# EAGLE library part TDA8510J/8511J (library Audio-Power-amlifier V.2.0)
The TDA8510J is an integrated class-B output amplifier in a 17-lead single-in-line (SIL) power package. It contains a 26 W Bridge-Tied Load (BTL) amplifier and 2 ´ 13 W Single-Ended (SE) amplifiers. The TDA8511J is an integrated class-B output amplifier in a 17-lead DIL-bent-SIL power package. It contains 4 ´ 13 W single-ended amplifiers.
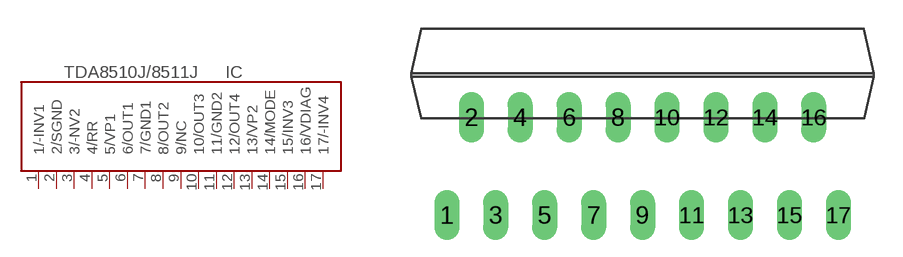
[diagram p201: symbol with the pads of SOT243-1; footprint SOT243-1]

Designator prefix IC

## TDA8510J/8511J  [SOT243-1]
1  1/-INV1  in
2  2/SGND  pwr
3  3/-NV2  in
4  4/RR  in
5  5/VP1  pwr
6  6/OUT1  out
7  7/GND1  pwr
8  8/OUT2  out
9  9/NC  nc
10  10/OUT3  out
11  11/GND2  pwr
12  12/OUT4  out
13  13/VP2  pwr
14  14/MODE  in
15  15/INV3  in
16  16/VDIAG  out
17  17/-INV4  in

## Footprint SOT243-1 (pad centres in mm)
DBS17P: plastic DIL-bent-SIL power package; 17 leads (lead length 7.7 mm)
drill 0.8 long: 1 -10.16,-5.08; 2 -8.89,0; 3 -7.62,-5.08; 4 -6.35,0; 5 -5.08,-5.08; 6 -3.81,0; 7 -2.54,-5.08; 8 -1.27,0; 9 0,-5.08; 10 1.27,0; 11 2.54,-5.08; 12 3.81,0; 13 5.08,-5.08; 14 6.35,0; 15 7.62,-5.08; 16 8.89,0; 17 10.17,-5.08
